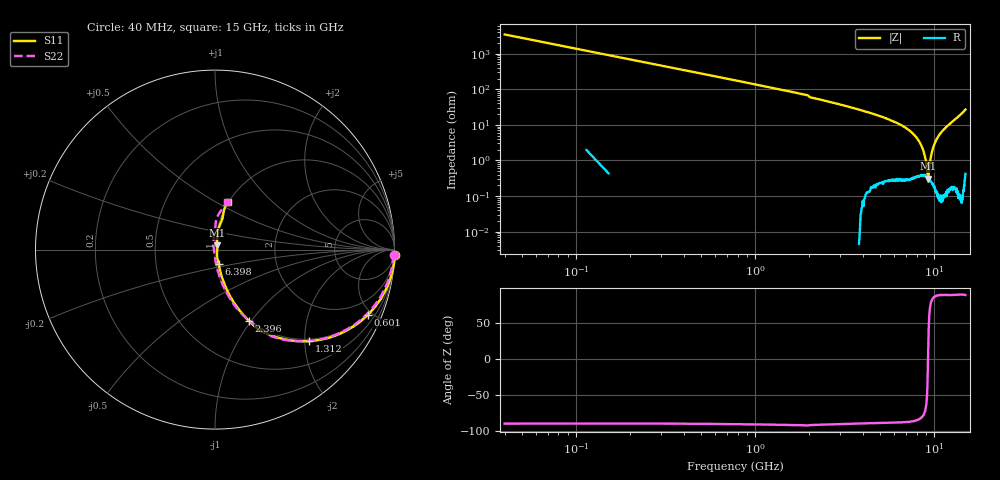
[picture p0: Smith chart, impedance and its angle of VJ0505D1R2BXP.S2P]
! VJ0505D1R2BXP
! MLCC placed on 25 mil thick microstrip substrate in series configuraton.
! DATE 06/29/2018  07:27
! CORRECTED  DATA
# GHz  S  MA  R  50.00
!  FREQ  S11M  S11A  S21M  S21A  S12M  S12A  S22M  S22A
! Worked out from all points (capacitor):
!   401 points, 40 MHz to 15 GHz, reference 50 ohm
!   read as one part in series: C = 1.14 pF near 114.8 MHz
!   lowest |Z| = 311 mohm at 9.278 GHz (marker M1)
!   series resonance near 9.276 GHz, so ESL is about 260 pH
!   S11 on the Smith chart (normalised r, x): 40 MHz: -9, -71; 601 MHz: 0.92, -4.69; 1.312 GHz: 0.96, -2.11; 2.396 GHz: 0.99, -0.97; 6.398 GHz: 1.03, -0.17; 15 GHz: 0.99, +0.57
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0.04  1.004 -1.6  0.02885 88.5  0.02906 88.2  0.9958 -1.6
0.1522  0.9977 -6.2  0.1088 83.8  0.1088 83.8  0.9898 -6.2
0.2644  0.9864 -10.7  0.1867 79.4  0.1868 79.5  0.9786 -10.6
0.414  0.9647 -16.4  0.2859 73.9  0.286 73.9  0.9564 -16.4
0.601  0.9251 -23.3  0.3992 67.5  0.3996 67.5  0.9183 -23.2
1.3116  0.7328 -44.1  0.7042 47.6  0.7045 47.7  0.7307 -44.2
2.097  0.5037 -61.6  0.8838 31.1  0.8842 31.1  0.4999 -60.5
2.3962  0.4397 -64.5  0.9098 27.2  0.9104 27.3  0.4407 -64.3
2.5458  0.4114 -65.8  0.9206 25.5  0.921 25.6  0.4136 -65.9
5.0516  0.1525 -75.9  0.9861 11.0  0.9864 11.0  0.1505 -80.6
6.398  0.08288 -76.1  0.9931 7.3  0.9936 7.4  0.08199 -86.0
7.52  0.03803 -72.3  0.9956 4.8  0.996 4.9  0.03847 -90.3
8.1184  0.01838 -51.7  0.9957 3.6  0.996 3.6  0.01727 -101.3
8.3802  0.0133 -24.3  0.9954 3.1  0.9958 3.1  0.009656 -122.5
8.5672  0.01236 3.6  0.9957 2.7  0.9956 2.8  0.006291 -164.8
8.6794  0.01341 19.7  0.9953 2.5  0.9958 2.5  0.006956 162.1
9.016  0.02001 50.1  0.9955 1.8  0.996 1.9  0.01538 119.3
9.2778  0.02709 63.2  0.9959 1.3  0.9965 1.4  0.02399 109.0
10.0258  0.0526 76.9  0.9962 -0.2  0.9968 -0.1  0.05197 98.8
10.886  0.082 80.2  0.9955 -2.0  0.9958 -1.9  0.08269 94.7
12.5316  0.1371 79.0  0.9883 -5.4  0.989 -5.3  0.1404 88.6
15  0.2745 74.7  0.9577 -13.9  0.9578 -13.9  0.2754 75.6
